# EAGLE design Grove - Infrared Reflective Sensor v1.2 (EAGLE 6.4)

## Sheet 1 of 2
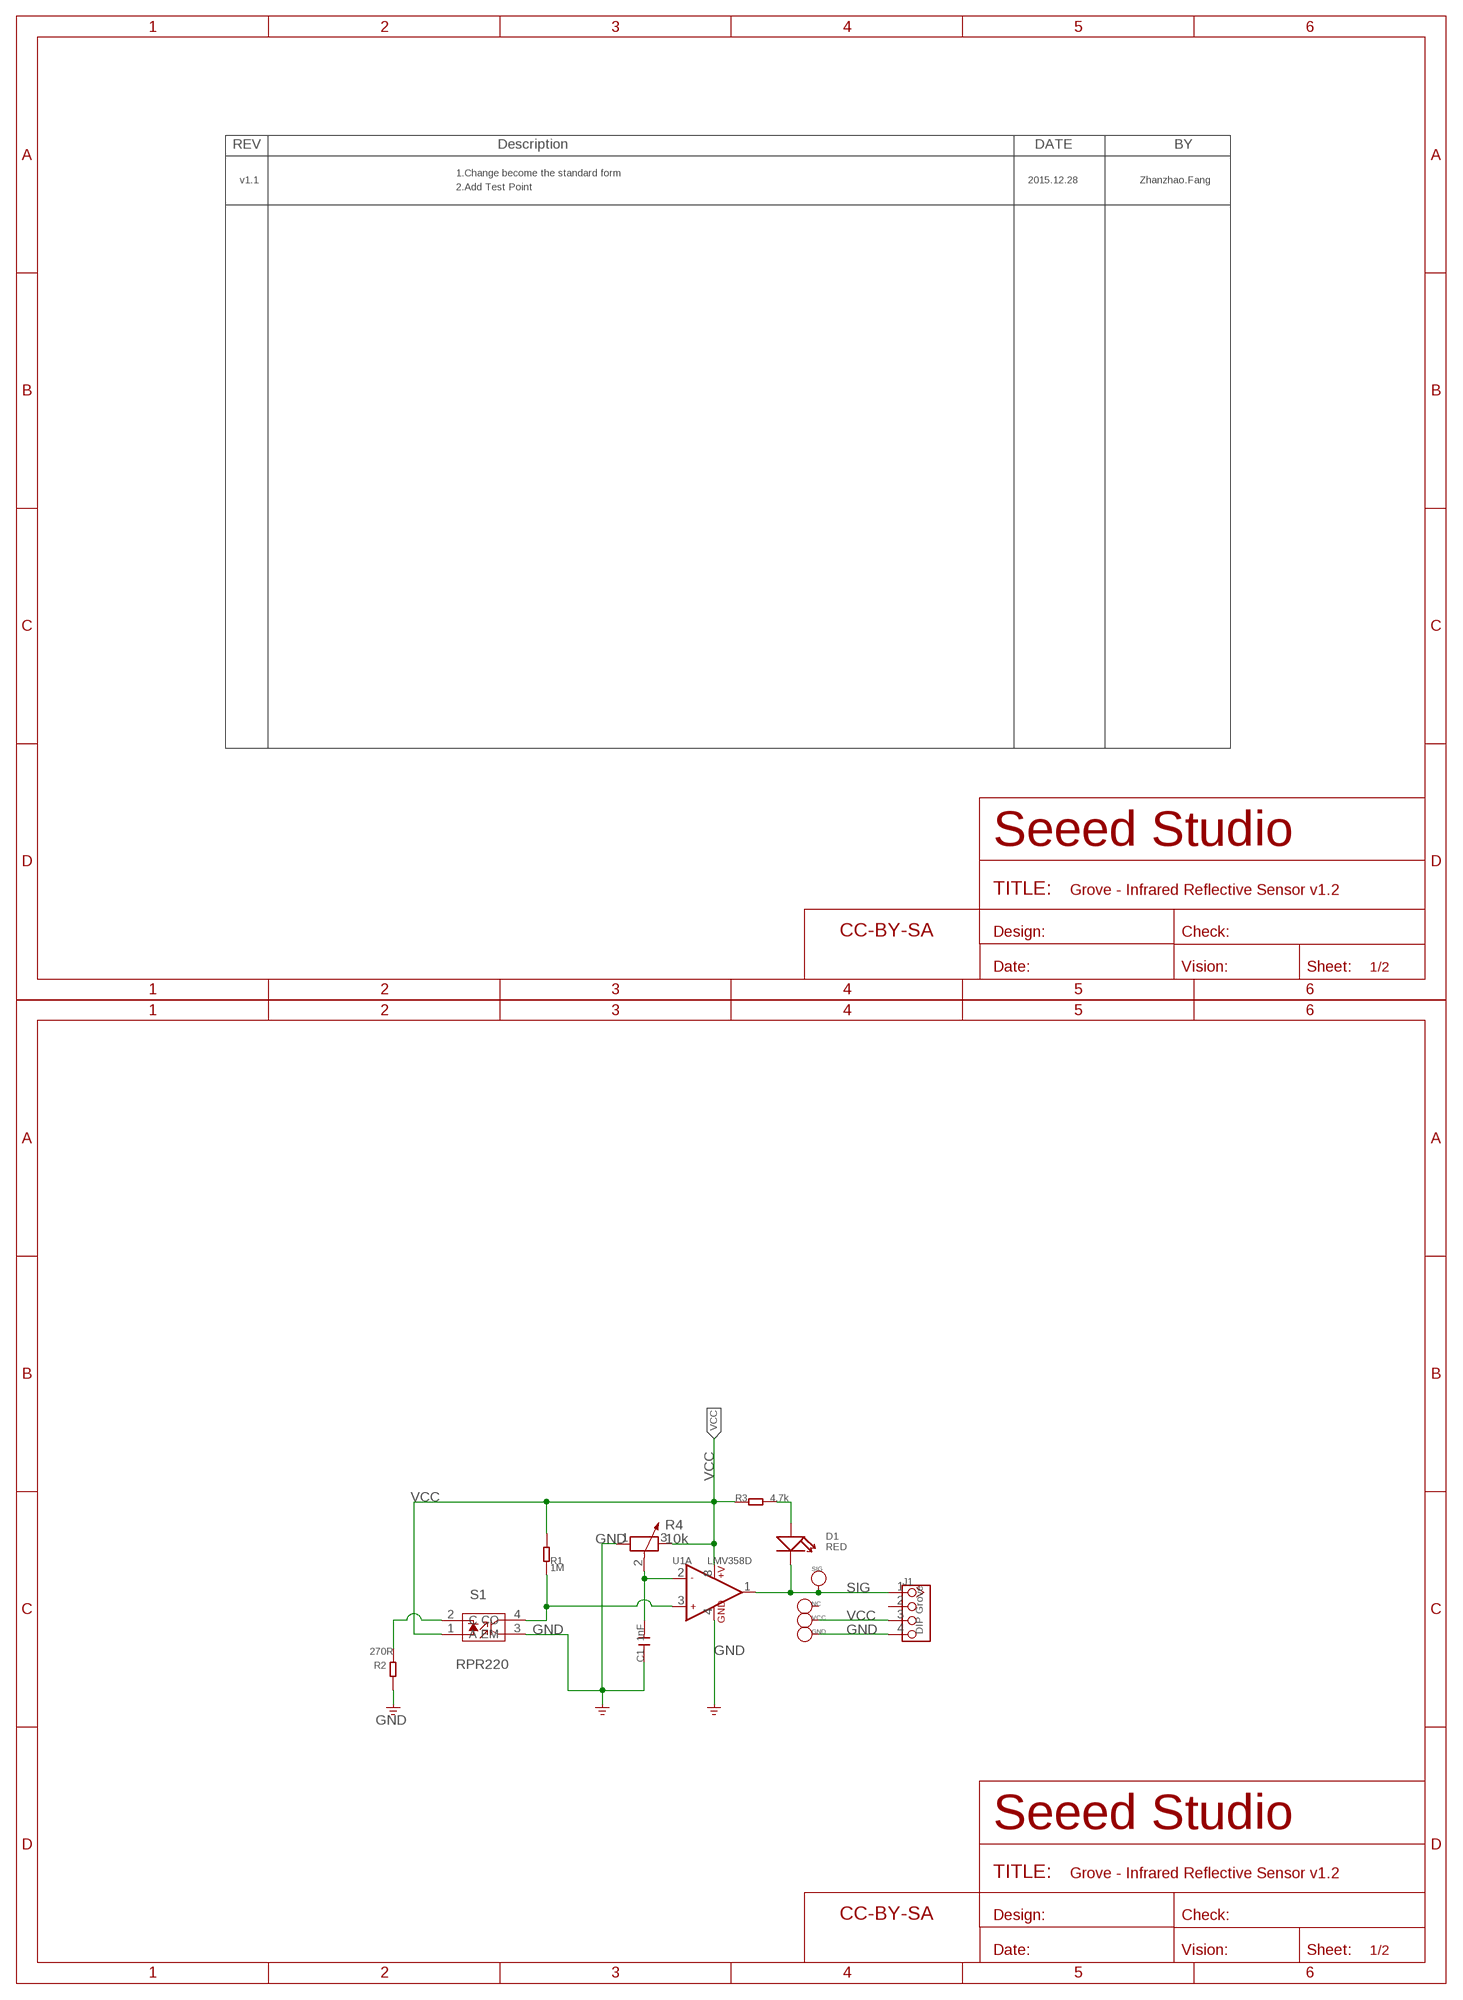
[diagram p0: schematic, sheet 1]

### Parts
C1  1nF  C-0603  [C0603]
D1  RED  LED'RIGHT'  [LED-SIDE-VIEW-0603-RIGHT]
FR1  DNP  SEEEDSTUDIO-OPEN-SCH-FRAME  [SEEEDSTUDIO-PCB-FRAME]
FR2  DNP  SEEEDSTUDIO-OPEN-SCH-FRAME  [SEEEDSTUDIO-PCB-FRAME]
GND  DNP  PAD-TEST-POINT'4545'  [TP_4545]
J1  DIP Grove  TWIG-4P-2.0-2.0  [4P-2.0]
NC  DNP  PAD-TEST-POINT'4545'  [TP_4545]
R1  1M  R-0603  [R0603]
R2  270R  R-0603  [R0603]
R3  4.7k  R-0603  [R0603]
R4  10k  R-POTENTIOMETER'RTRIM3214W'  [3P-SMD-SQUA-4.6X3.7]
S1  RPR220  SENSOR-OPTICAL-RPR-220  [SNR4-6.4X4.9X6.5MM]
SIG  DNP  PAD-TEST-POINT'4545'  [TP_4545]
U1  LMV358D  [SO08]
VCC  DNP  PAD-TEST-POINT'4545'  [TP_4545]

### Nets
GND: C1.1 GND.T J1.4 R2.1 R4.1 S1.3(EM) U1.4(A:GND) ; supply symbol labelled GND_POWER
N$1: C1.2 R4.2 U1.2(A:-IN1)
N$2: R1.1 S1.4(CO) U1.3(A:+IN1)
N$5: R2.2 S1.2(C)
N$12: D1.1(+) R3.2
SIG: D1.2(-) J1.1 SIG.T U1.1(A:OUT1)
VCC: J1.3 R1.2 R3.1 R4.3 S1.1(A) U1.8(A:+V) VCC.T
Unconnected: J1.2 NC.T U1.5(B:+IN2) U1.6(B:-IN2) U1.7(B:OUT2)

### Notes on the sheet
- 1.Change become the standard form
- v1.1 | 2015.12.28 | Zhanzhao.Fang
- 2.Add Test Point

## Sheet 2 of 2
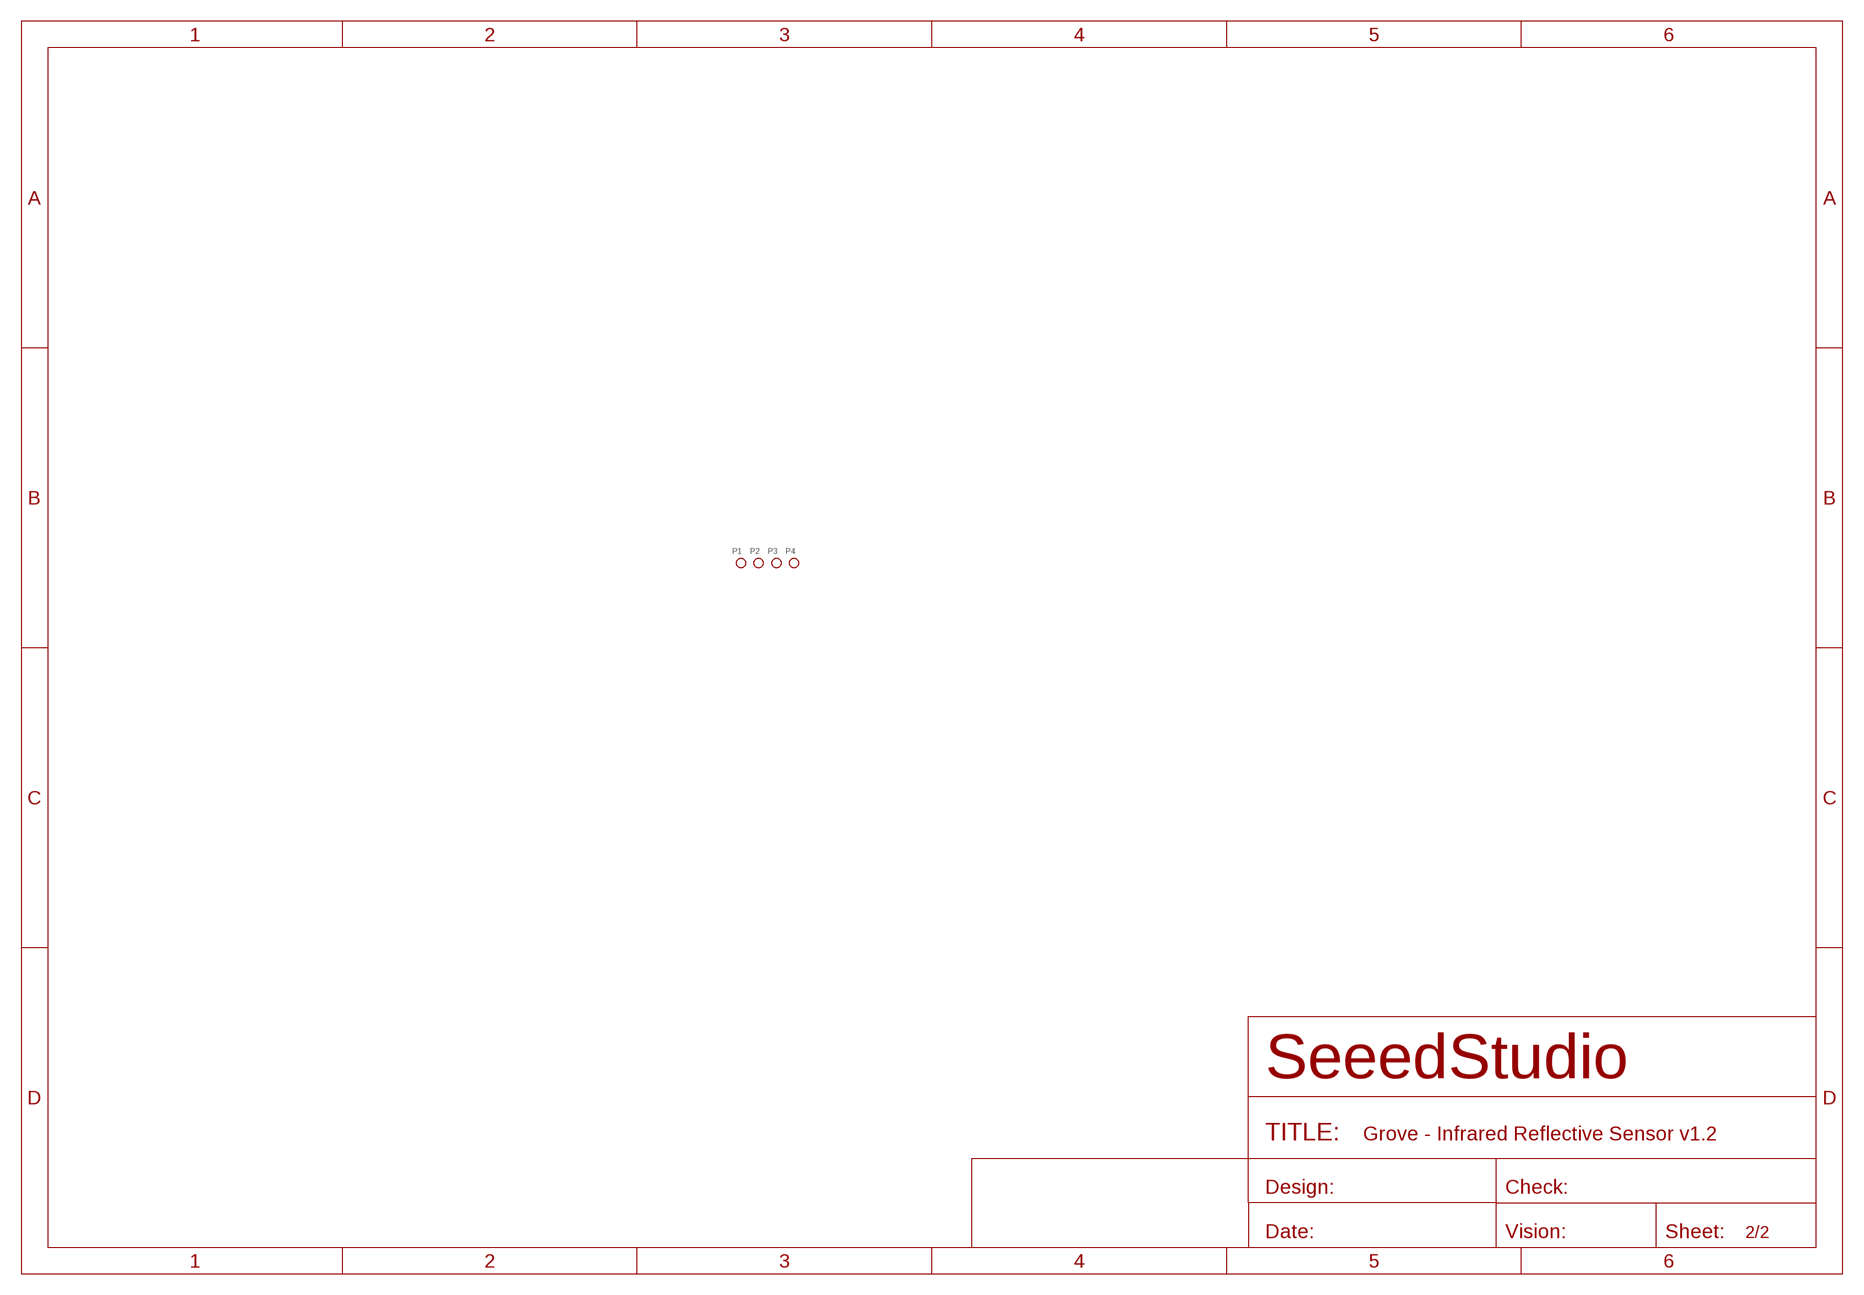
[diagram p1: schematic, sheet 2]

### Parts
P1  DNP  PAD-MARK  [ROUND-MARK-1.0]
P2  DNP  PAD-MARK  [ROUND-MARK-1.0]
P3  DNP  PAD-MARK  [ROUND-MARK-1.0]
P4  DNP  PAD-MARK  [ROUND-MARK-1.0]

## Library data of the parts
C1 = Discrete:C*: Ceramic Capacitors
D1 = Discrete-new:LED
FR1 FR2 = moudle-new:SEEEDSTUDIO-OPEN-SCH-FRAME
GND NC SIG VCC = Discrete:PAD-TEST-POINT; PARTNO: DNP
J1 = Connector:TWIG-4P-2.0
P1-P4 = Discrete:PAD-MARK; PARTNO: DNP
R1-R3 = Discrete:R*
R4 = Discrete:R-POTENTIOMETER*: Potentiometer
S1 = Discrete-new:SENSOR-OPTICAL-RPR-220: 314020002
U1 = IC:LMV358: General purpose LOW Voltage, Rail-to-Rail Output Amplifiers http://www.fairchildsemi.com/ds/LM/LMV358.pdf

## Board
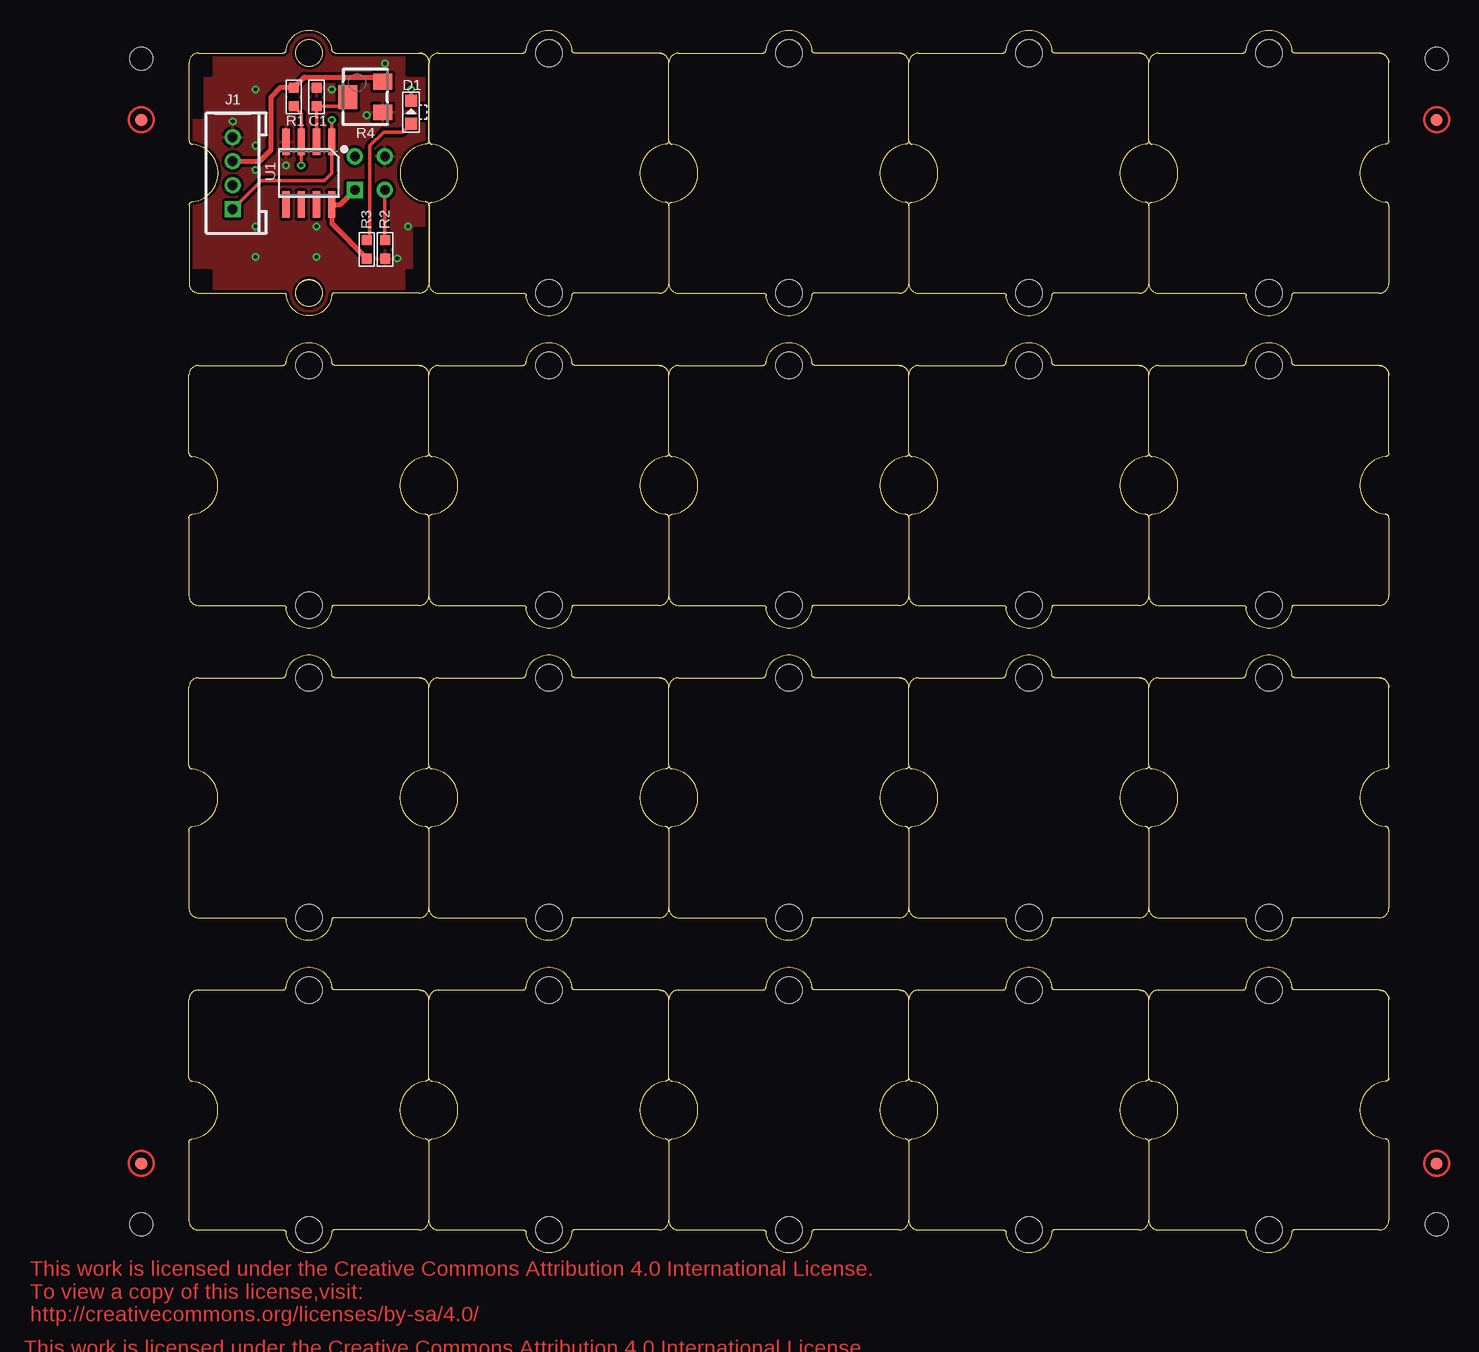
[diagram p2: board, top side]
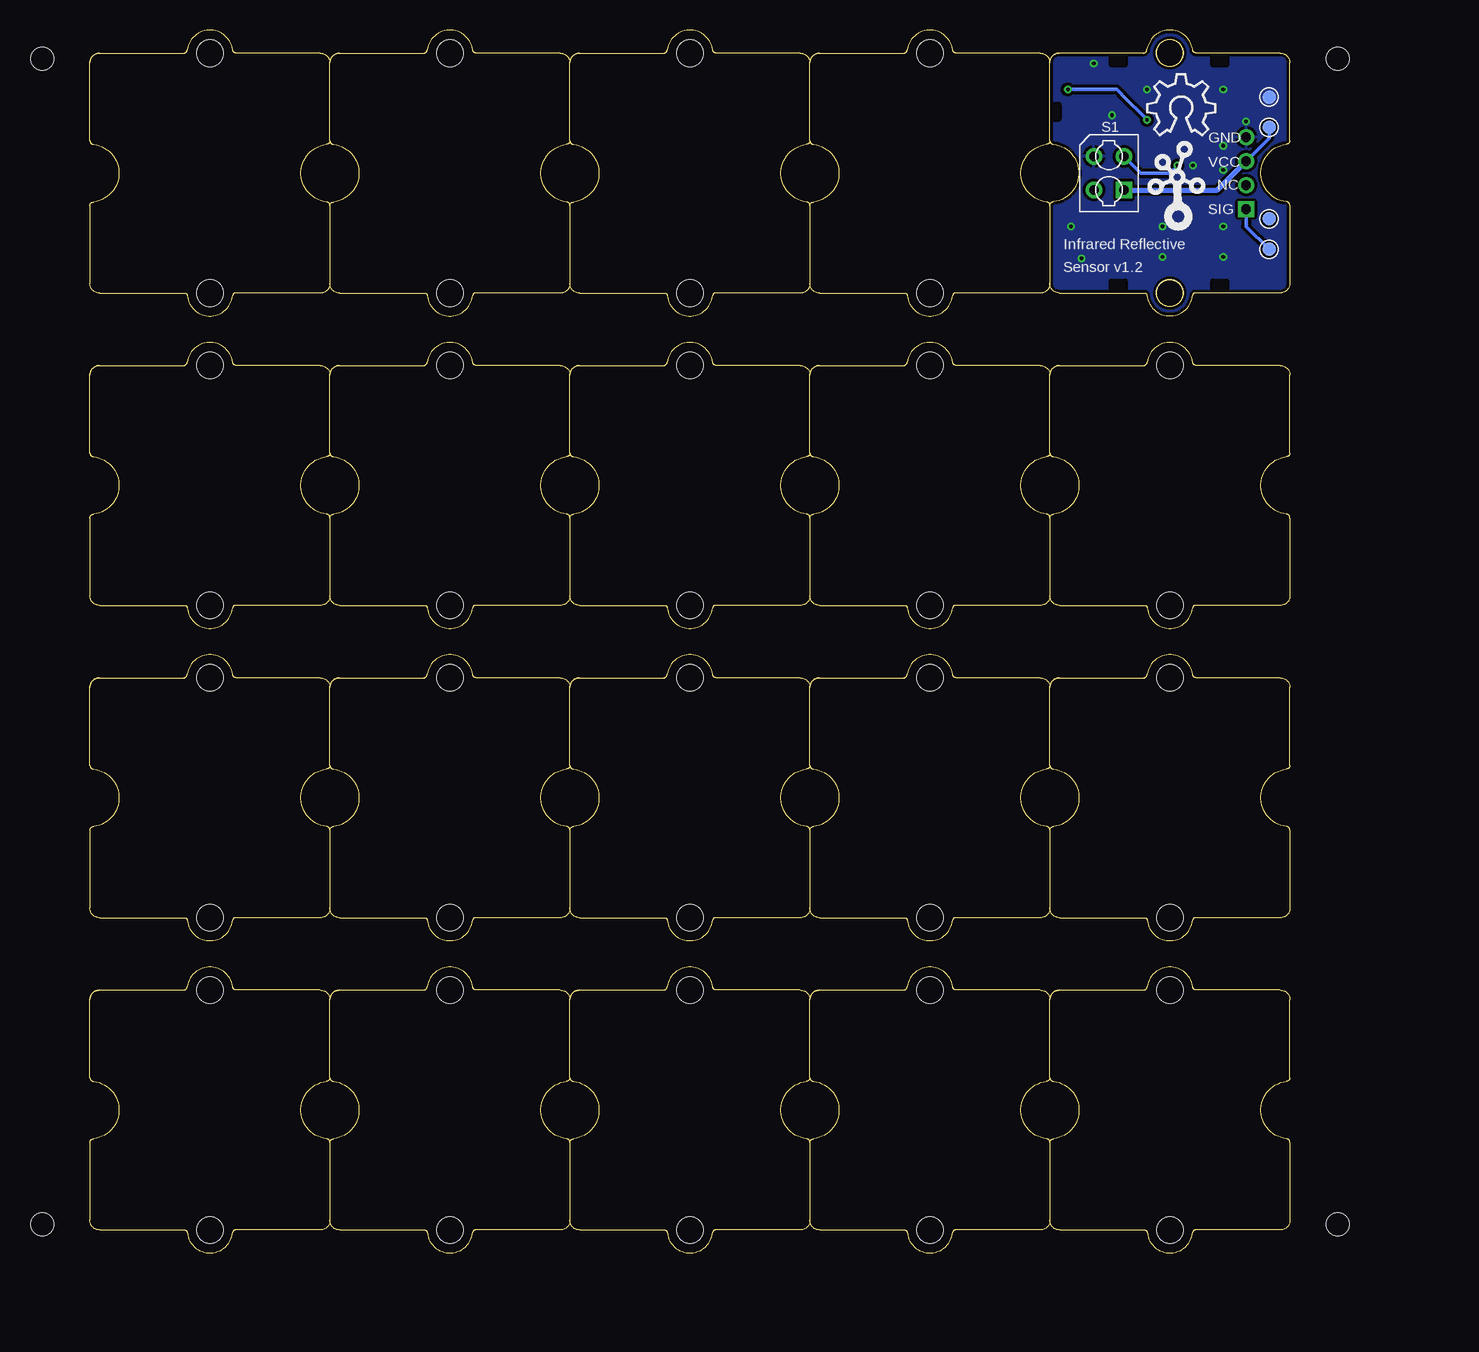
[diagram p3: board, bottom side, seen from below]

Size 100 x 101.95 mm. Coordinates in mm from the lower left corner, seen from the top.
Copper layers (1*16): Top 0.035mm / dielectric 1.5mm / Bottom 0.035mm
Design rules "default": minimum track width 6mil, minimum drill 12mil, track to track 6mil, track to pad 6mil, pad to pad 6mil, via to via 6mil, smd to smd 0mil, copper to edge 10mil, drill to drill 10mil, minimum pad ring 10mil, minimum via ring 6mil, stop-mask expansion 2mil, vias tented up to drill 100mil, thermal gap 10mil
Holes 1.91 mm at -3.97,2.38 -3.97,99.54 103.98,99.54 103.98,2.38
tRestrict: area 19.3,94.5 to 19.8,95.7
bRestrict: area 19.3,94.5 to 19.8,95.7

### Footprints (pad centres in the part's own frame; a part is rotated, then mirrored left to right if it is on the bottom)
C0603 = smd 0.889 x 0.889: 1 -0.762,0; 2 0.762,0
LED-SIDE-VIEW-0603-RIGHT = smd 1 x 1: 1 0,-0.95; 2 0,0.95
TP_4545 = smd 1.143 x 1.143: T 0,0
4P-2.0 = drill 0.8 pad 1.27 square: 1 -3,0 | drill 0.8 pad 1.27: 2 -1,0; 3 1,0; 4 3,0
ROUND-MARK-1.0 = smd 1.016 x 1.016: P$1 0,0
R0603 = smd 0.889 x 0.889: 1 -0.762,0; 2 0.762,0
3P-SMD-SQUA-4.6X3.7 = smd 1.3 x 1.6: 1 -1.275,-1.45; 3 1.275,-1.45 | smd 2 x 1.6: 2 0,1.45
SNR4-6.4X4.9X6.5MM = drill 0.8 pad 1.35 square: 1 -1.4,-1.25 | drill 0.8 pad 1.35: 2 -1.4,1.25; 3 1.4,1.25; 4 1.4,-1.25
SO08 = smd 0.61 x 2.21: 1 -1.905,-2.616; 2 -0.635,-2.616; 3 0.635,-2.616; 4 1.905,-2.616; 5 1.905,2.616; 6 0.635,2.616; 7 -0.635,2.616; 8 -1.905,2.616
1U-DIM-W/-DRILL = hole 2.2: 0,-10; 0,10
GROVE-1X1-TEST-PLATFORM = hole 2.2: 9.987,0.013; -10.013,0.013

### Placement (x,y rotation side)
C1  10.63,96.36 270 top
D1  18.51,95.09 0 top
FR1  not placed on the board
FR2  not placed on the board
GND  1.74,96.36 0 bottom
J1  3.65,90.01 90 top
NC  1.74,86.2 0 bottom
P1  not placed on the board
P2  not placed on the board
P3  not placed on the board
P4  not placed on the board
R1  8.73,96.36 90 top
R2  16.35,83.66 90 top
R3  14.83,83.66 90 top
R4  14.7,96.36 90 top
S1  15.08,90.01 90 bottom
SIG  1.74,83.66 0 bottom
U1  10,90.01 180 top
U$4  [TWIGLOGO]  9.37,86.2 0 bottom
U$5  [OSHW_8X200_NOTEXT]  11.9,93.19 0 bottom
U$7  [1U-DIM-W/-DRILL]  30,90.01 0 top
U$8  [1U-DIM-W/-DRILL]  50,90.01 0 top
U$9  [1U-DIM-W/-DRILL]  70,90.01 0 top
U$10  [1U-DIM-W/-DRILL]  90,90.01 0 top
U$11  [1U-DIM-W/-DRILL]  30,63.98 0 top
U$12  [1U-DIM-W/-DRILL]  50,63.98 0 top
U$13  [1U-DIM-W/-DRILL]  70,63.98 0 top
U$14  [1U-DIM-W/-DRILL]  90,63.98 0 top
U$15  [1U-DIM-W/-DRILL]  10,63.98 0 top
U$16  [1U-DIM-W/-DRILL]  30,37.94 0 top
U$17  [1U-DIM-W/-DRILL]  50,37.94 0 top
U$18  [1U-DIM-W/-DRILL]  70,37.94 0 top
U$19  [1U-DIM-W/-DRILL]  90,37.94 0 top
U$20  [1U-DIM-W/-DRILL]  10,37.94 0 top
U$21  [1U-DIM-W/-DRILL]  30,11.91 0 top
U$22  [1U-DIM-W/-DRILL]  50,11.91 0 top
U$23  [1U-DIM-W/-DRILL]  70,11.91 0 top
U$24  [1U-DIM-W/-DRILL]  90,11.91 0 top
U$25  [1U-DIM-W/-DRILL]  10,11.91 0 top
U$29  [GROVE-1X1-TEST-PLATFORM]  10,90.01 270 top
VCC  1.74,93.82 0 bottom

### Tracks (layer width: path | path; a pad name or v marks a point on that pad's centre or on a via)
GND  (via drill 0.3 pad 0.64)
  other vias: 8.1,90.65 11.9,97 18.26,85.57 5.55,97 5.55,92.3 10.63,85.57 5.55,85.57 14.83,94.84 17.37,82.9 10.63,83.03 5.55,83.03 3.65,94.33 16.35,99.16 5.55,90.27
  pour Bottom (isolate 0.254): -0.79,102.71 20.8,102.71 20.8,77.95 -0.79,77.95
  pour Top (isolate 0.254): -0.79,102.71 20.8,102.71 20.8,77.95 -0.79,77.95
N$1
  Top 0.305: U1.2 C1.2 12.49,95.6 R4.2
N$2  (via drill 0.3 pad 0.64)
  Top 0.305: R1.1 9.37,94.97 U1.3 v9.37,90.65
  Bottom 0.305: v9.37,90.65 10,90.01 12.43,90.01 S1.4
N$5
  Top 0.305: S1.2 16.33,84.57 16.35,84.55 R2.2
N$12
  Top 0.305: R3.2 15.08,84.68 15.08,92.3 16.22,93.44 17.81,93.44 D1.1
SIG  (via drill 0.3 pad 0.64)
  Top 0.305: J1.1 6.02,89.38 11.27,89.38 11.9,90.01 U1.1 v11.9,94.46 | D1.2 v18.51,97
  Bottom 0.305: J1.1 3.65,85.57 SIG.T | v11.9,94.46 14,96.55 14.06,96.62 14.45,97 v18.51,97
VCC
  Top 0.406: 16.35,98.01 16.35,97.89 16.22,97.76 16.34,97.64 R4.3 15.77,98.01 9.62,98.01 R1.2 7.59,97.13 6.83,96.36 6.83,91.92 5.92,91.01 J1.3 | S1.1 12.61,87.4 U1.8 11.9,85.82 R3.1
  Bottom 0.305: VCC.T 1.74,92.92 J1.3
  Bottom 0.406: S1.1 6.05,88.61 J1.3

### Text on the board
bPlace: GND | VCC | NC | SIG | Infrared Reflective | Sensor v1.2
bDocu: GND | VCC | NC | SIG

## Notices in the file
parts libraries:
moudle-new: This work is licensed under the Creative Commons Attribution 4.0 International License.
To view a copy of this license,visit:
http://creativecommons.org/licenses/by-sa/4.0
moudle-new: CC-BY-SA
